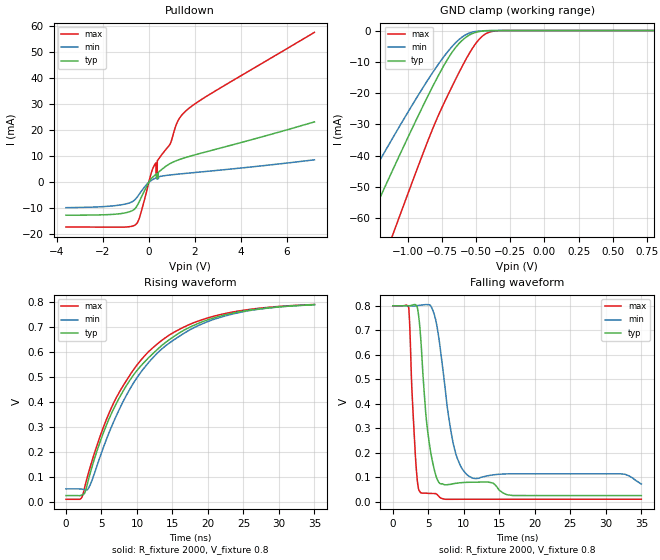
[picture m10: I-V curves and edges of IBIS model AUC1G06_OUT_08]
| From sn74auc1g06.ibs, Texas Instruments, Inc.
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[Model]   AUC1G06_OUT_08
Model_type  Open_drain
Enable   Active-Low
Vref =   0
Rref =   2000
Cref =   15p
Vmeas =   0.4
| variable   typ   min   max
C_comp   2.80pF   2.35pF   3.27pF
| C_pulldown   4.29pF   3.36pF   5.30pF
| C_tri-state   2.80pF   2.35pF   3.27pF
[Temperature Range]   40   100   -40
| Ambient temperature   25   85   -40
[Voltage range]   0.8   0.8   0.8
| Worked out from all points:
|   slope of the pulldown table from 0 to 0.12 V, typ, clamps not added: 77.1 ohm
|   GND clamp passes 1 mA (typ) near -0.53 V on its own axis
|   rising waveform, R_fixture 2000, V_fixture 0.8: 20-80 % time 9.86ns typ, 9.84ns min, 9.25ns max; typ from 0.025 V to 0.789 V
|   falling waveform, R_fixture 2000, V_fixture 0.8: 20-80 % time 1.49ns typ, 2.12ns min, 747ps max; typ from 0.8 V to 0.025 V
[GND Clamp]
| AUC1G06_OUT_08
|   Voltage   I(typ)   I(min)   I(max)
-3.6V     -288.1mA   -237.2mA   -357.2mA
-1.5V     -82.06mA   -64.54mA   -111.6mA
-1.325V   -65.12mA   -50.81mA   -90.87mA
-1.28V    -60.78mA   -47.32mA   -85.53mA
-1.115V   -45.05mA   -34.73mA   -65.91mA
-1.08V    -41.75mA   -32.1mA    -61.76mA
-835mV    -19.39mA   -14.59mA   -33.3mA
-690mV    -7.898mA   -5.836mA   -19.16mA
-570mV    -2.027mA   -1.223mA   -8.88mA
-445mV    -148.6uA   -75.24uA   -1.502mA
-310mV    -2.967uA   -2.428uA   -23.93uA
800mV     186.8pA    342.6pA    147.7pA
[Pulldown]
| AUC1G06_OUT_08
|   Voltage   I(typ)   I(min)   I(max)
-3.6V     -12.63mA   -9.733mA   -17.19mA
-570mV    -9.824mA   -6.355mA   -16.25mA
-385mV    -6.858mA   -4.174mA   -13.02mA
190mV     2.176mA    1.163mA    5.632mA
310mV     3.079mA    1.693mA    7.502mA
315mV     3.117mA    1.714mA    2.469mA
365mV     1.692mA    1.285mA    2.781mA
370mV     1.723mA    1.302mA    8.254mA
925mV     7.223mA    2.844mA    14.73mA
1.215V    8.403mA    3.118mA    22.65mA
1.49V     9.255mA    3.359mA    26.44mA
7.2V      23.27mA    8.676mA    57.72mA
[Ramp]
| AUC1G06_OUT_08
| variable   typ   min   max
dV/dt_r   0.46/9.87E-09   0.45/9.85E-09   0.47/9.25E-09
dV/dt_f   0.47/1.54E-09   0.44/2.25E-09   0.48/7.70E-10
R_load = 2000
[Rising Waveform]
| AUC1G06_OUT_08
R_fixture =   2000
C_fixture =   0
L_fixture =   0
V_fixture =   0.8
V_fixture_min = 0.8
V_fixture_max = 0.8
|   Time   V(typ)   V(min)   V(max)
0s        25.46mV    52.25mV    10.6mV
2.16ns    26.78mV    51.51mV    15.41mV
2.65ns    36mV       48.56mV    60.1mV
3.145ns   86.62mV    53.51mV    113.2mV
5.205ns   271.7mV    212.8mV    293.6mV
7.485ns   415.1mV    368.9mV    437.8mV
10.09ns   529.1mV    500.9mV    551.1mV
13.29ns   621.3mV    607.2mV    642.3mV
21.87ns   745mV      740mV      750.7mV
34.99ns   789.2mV    790mV      790.4mV
[Falling Waveform]
| AUC1G06_OUT_08
R_fixture =   2000
C_fixture =   0
L_fixture =   0
V_fixture =   0.8
V_fixture_min = 0.8
V_fixture_max = 0.8
|   Time   V(typ)   V(min)   V(max)
0s        800mV      800mV      800mV
2.235ns   800.1mV    799.8mV    793.6mV
2.68ns    802.4mV    799.2mV    462.3mV
3.205ns   804.1mV    799.6mV    175.8mV
3.935ns   664.5mV    802.6mV    37.07mV
4.82ns    309.1mV    804.7mV    34.96mV
6.115ns   102.4mV    732mV      32.5mV
8.44ns    73.33mV    247.3mV    10.32mV
10.54ns   79.66mV    108.2mV    10.59mV
34.99ns   25.47mV    72.43mV    10.6mV
